(* Logix 5000 AddOnInstructionDefinition export FMQ_AOI_4P; software revision 33.00 *)

ADD_ON_INSTRUCTION FMQ_AOI_4P   (* revision 1.0, vendor PM Controls *)
// Anderson-Negele Flow Sensor
// Revision note:
// psm
VAR_OUTPUT
   IOLink_Mode : BOOL; {access Read Only, visible}
   Device_Not_Connected : BOOL; {access Read Only, visible}
END_VAR
VAR_IN_OUT
   Input : INT[123]; {required}
END_VAR
VAR_INPUT
   Port_Process_Data_Size : INT := 4;
   Port_Number : INT; {visible}
END_VAR
VAR_OUTPUT
   Vendor_ID : INT; {access Read Only, visible}
   Device_ID : DINT; {access Read Only, visible}
   Invalid_Data : BOOL; {access Read Only, visible}
   Volume : REAL; {access Read Only, visible}
   Flow_Rate : REAL; {access Read Only, visible}
   Total_Volume : REAL; {access Read Only, visible}
END_VAR
VAR
   StatusFlgs_Offset : INT; {access None}
   RealPort_Num : INT; {access None}
   Process_Offset : INT; {access None}
   Offset_StatusFlgs : INT; {access None}
   Offset_Address : INT; {access None}
   Data_Size : INT; {access None}
   VolumeDINT : DINT; {access None}
   Total_Volume_INT : INT[2]; {access None}
   Total_Volume_DINT : DINT; {access None}
   Flow_Rate_INT : INT[2]; {access None}
   Flow_RateDINT : DINT; {access None}
   Volume_INT : INT[2]; {access None}
END_VAR

ROUTINE Logic   (* ladder *)
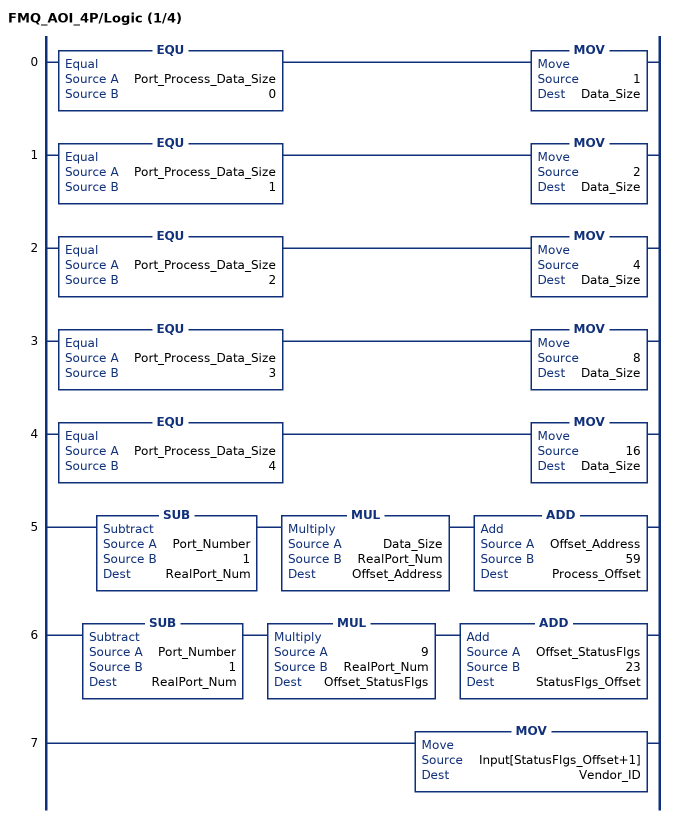
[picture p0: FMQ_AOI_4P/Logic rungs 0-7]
   0: EQU(Port_Process_Data_Size,0)MOV(1,Data_Size);
   1: EQU(Port_Process_Data_Size,1)MOV(2,Data_Size);
   2: EQU(Port_Process_Data_Size,2)MOV(4,Data_Size);
   3: EQU(Port_Process_Data_Size,3)MOV(8,Data_Size);
   4: EQU(Port_Process_Data_Size,4)MOV(16,Data_Size);
   5: SUB(Port_Number,1,RealPort_Num)MUL(Data_Size,RealPort_Num,Offset_Address)ADD(Offset_Address,59,Process_Offset);
   6: SUB(Port_Number,1,RealPort_Num)MUL(9,RealPort_Num,Offset_StatusFlgs)ADD(Offset_StatusFlgs,23,StatusFlgs_Offset);
   7: MOV(Input[StatusFlgs_Offset+1],Vendor_ID);
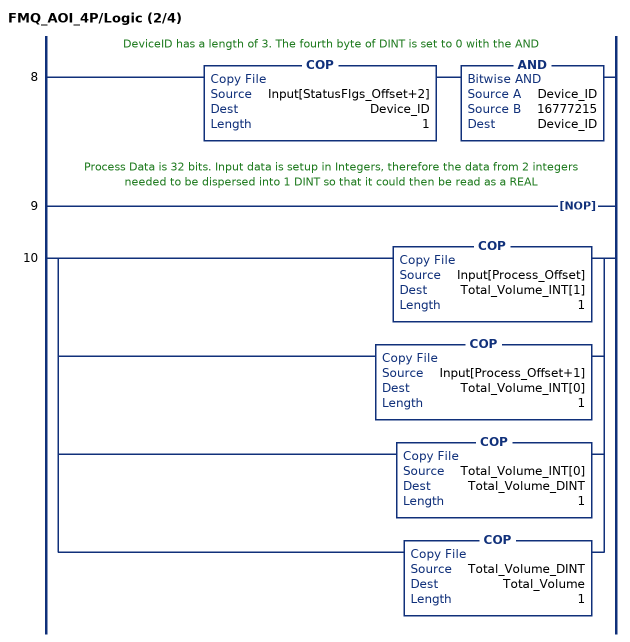
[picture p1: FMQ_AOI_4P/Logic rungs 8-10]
   // DeviceID has a length of 3. The fourth byte of DINT is set to 0 with the AND
   8: COP(Input[StatusFlgs_Offset+2],Device_ID,1)AND(Device_ID,16777215,Device_ID);
   // Process Data is 32 bits. Input data is setup in Integers, therefore the data from 2 integers needed to be dispersed into 1 DINT so that it could then be read as a REAL
   9: NOP();
   10: [COP(Input[Process_Offset],Total_Volume_INT[1],1) ,COP(Input[Process_Offset+1],Total_Volume_INT[0],1) ,COP(Total_Volume_INT[0],Total_Volume_DINT,1) ,COP(Total_Volume_DINT,Total_Volume,1) ];
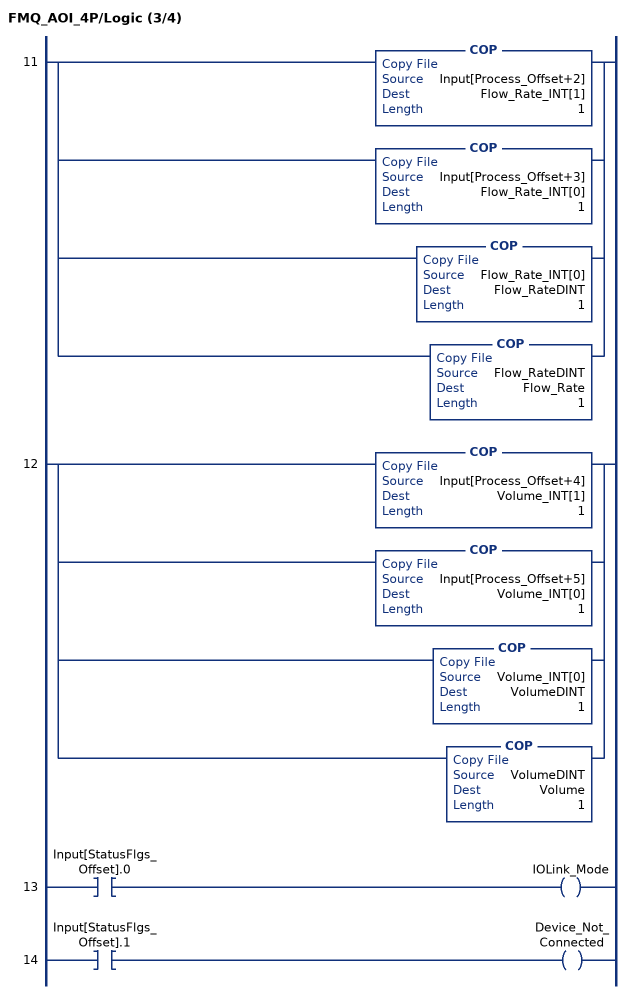
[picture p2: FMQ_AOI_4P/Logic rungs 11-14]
   11: [COP(Input[Process_Offset+2],Flow_Rate_INT[1],1) ,COP(Input[Process_Offset+3],Flow_Rate_INT[0],1) ,COP(Flow_Rate_INT[0],Flow_RateDINT,1) ,COP(Flow_RateDINT,Flow_Rate,1) ];
   12: [COP(Input[Process_Offset+4],Volume_INT[1],1) ,COP(Input[Process_Offset+5],Volume_INT[0],1) ,COP(Volume_INT[0],VolumeDINT,1) ,COP(VolumeDINT,Volume,1) ];
   13: XIC(Input[StatusFlgs_Offset].0)OTE(IOLink_Mode);
   14: XIC(Input[StatusFlgs_Offset].1)OTE(Device_Not_Connected);
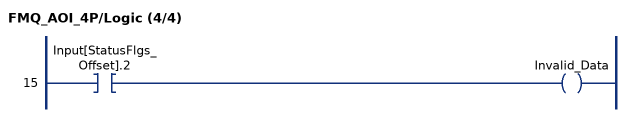
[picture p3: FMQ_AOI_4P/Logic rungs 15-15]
   15: XIC(Input[StatusFlgs_Offset].2)OTE(Invalid_Data);
END_ROUTINE
END_ADD_ON_INSTRUCTION
